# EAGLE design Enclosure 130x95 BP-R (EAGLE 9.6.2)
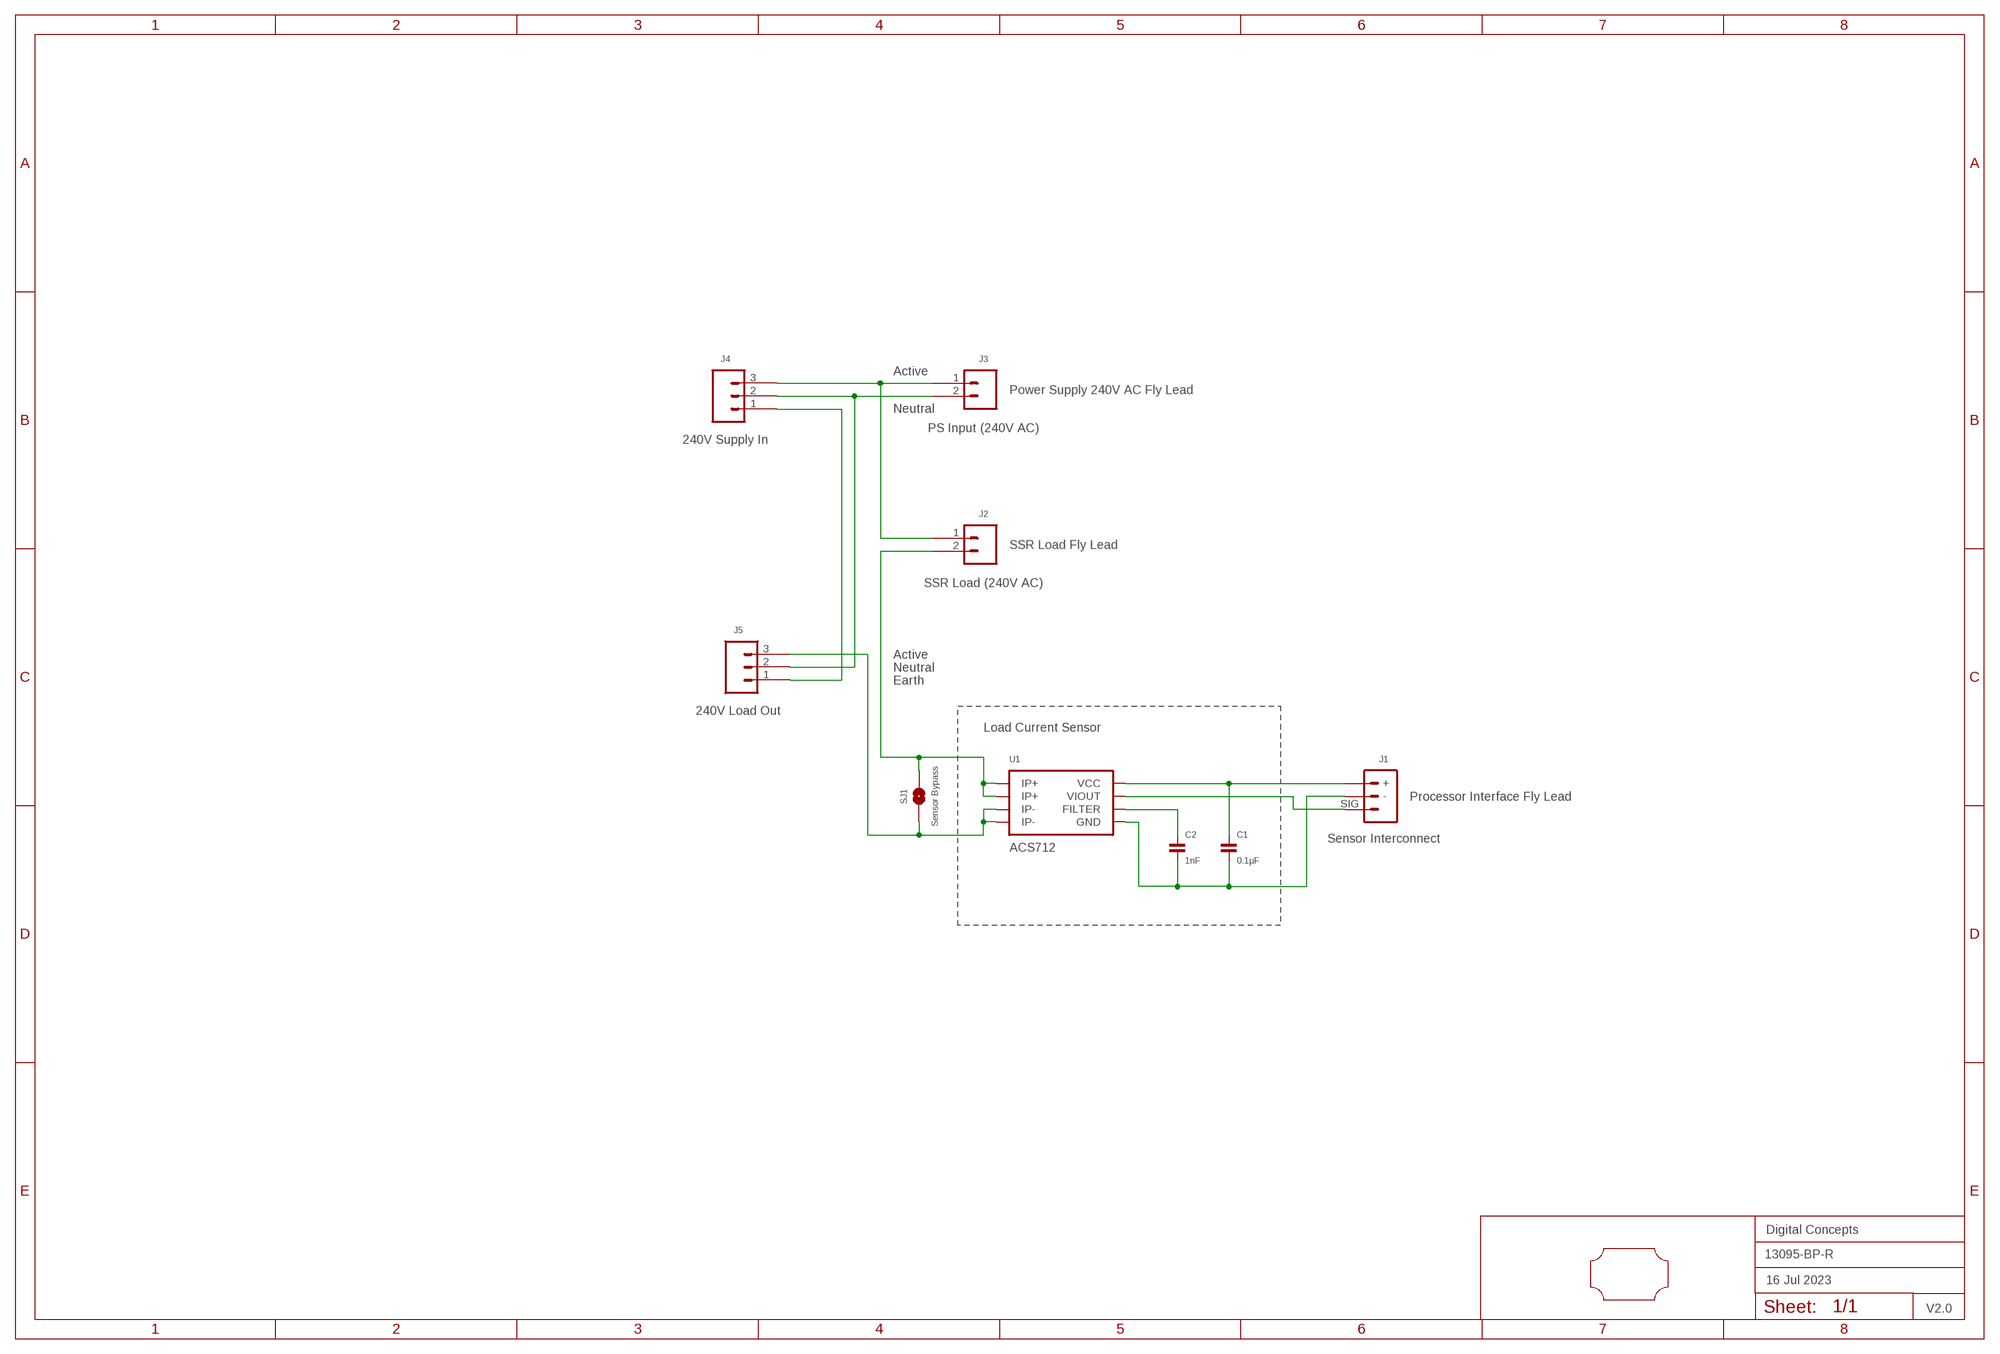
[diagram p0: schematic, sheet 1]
FRAME2 (A3L-LOC): DATE: 16 Jul 2023; OWNER: Digital Concepts; TITLE: 13095-BP-R; VERSION: V2.0

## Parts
C1  0.1µF  CAPACITOR-0805  [C0805]
C2  1nF  CAPACITOR-0805  [C0805]
J1  Sensor Interconnect  JST-PH2.0-3-HORIZONTAL  [JST-PH2.0-3-HORIZONTAL-SIG]
J2  SSR Load (240V AC)  TERMINAL_SCREW_2P_VERTICAL  [TERMINAL-SCREW-2P]
J3  PS Input (240V AC)  JST-XH2.54-2-HORIZONTAL  [JST-XH2.4-2-HORIZONTAL]
J4  240V Supply In  TERMINAL_SCREW_3P_VERTICAL  [TERMINAL-SCREW-3P]
J5  240V Load Out  TERMINAL_SCREW_3P_VERTICAL  [TERMINAL-SCREW-3P]
SJ1  Sensor Bypass  SJ  [SJ]
U1  ACS712  [SOIC-8]
U$1  PCB-OUTLINE-130X95-MAX-RC-H2  [PROTO-130X95-OUTLINE-MAX-RC-H2]

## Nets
ACTIVE_IN: J2.1 J3.1 J4.3
ACTIVE_OUT: J2.2 SJ1.2 U1.P$1(IP+) U1.P$2(IP+)
EARTH: J4.1 J5.1
N$19: J5.3 SJ1.1 U1.P$3(IP-) U1.P$4(IP-)
N$20: C1.2 C2.2 J1.- U1.P$5(GND)
N$22: J1.SIG U1.P$7(VIOUT)
N$23: C1.1 J1.+ U1.P$8(VCC)
N$24: C2.1 U1.P$6(FILTER)
NEUTRAL: J3.2 J4.2 J5.2

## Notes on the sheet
- Active
- Power Supply 240V AC Fly Lead
- Neutral
- SSR Load Fly Lead
- Active
- Neutral
- Earth
- Load Current Sensor
- Processor Interface Fly Lead

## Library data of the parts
C1 C2 = digitalconcepts:CAPACITOR-0805: 0805 Capacitor
J1 = digitalconcepts:JST-PH2.0-3-HORIZONTAL: PH2.0 3P Horizontal Connector
J2 = digitalconcepts:TERMINAL_SCREW_2P_VERTICAL: PCB Mount Screw-Type Terminal 2P
J3 = digitalconcepts:JST-XH2.54-2-HORIZONTAL: XH2.54 2P Horizontal Connector
J4 J5 = digitalconcepts:TERMINAL_SCREW_3P_VERTICAL: PCB Mount Screw-Type Terminal 3P
SJ1 = digitalconcepts:SJ: Solder Jumper
U1 = digitalconcepts:ACS712: ACS712 Hall-Effect-Based Linear Current Sensor IC
U$1 = digitalconcepts:PCB-OUTLINE-130X95-MAX-RC-H2: PCB Eagle Max-Right-Cropped outline for 130 x 95 enclosure (Horizontal format)

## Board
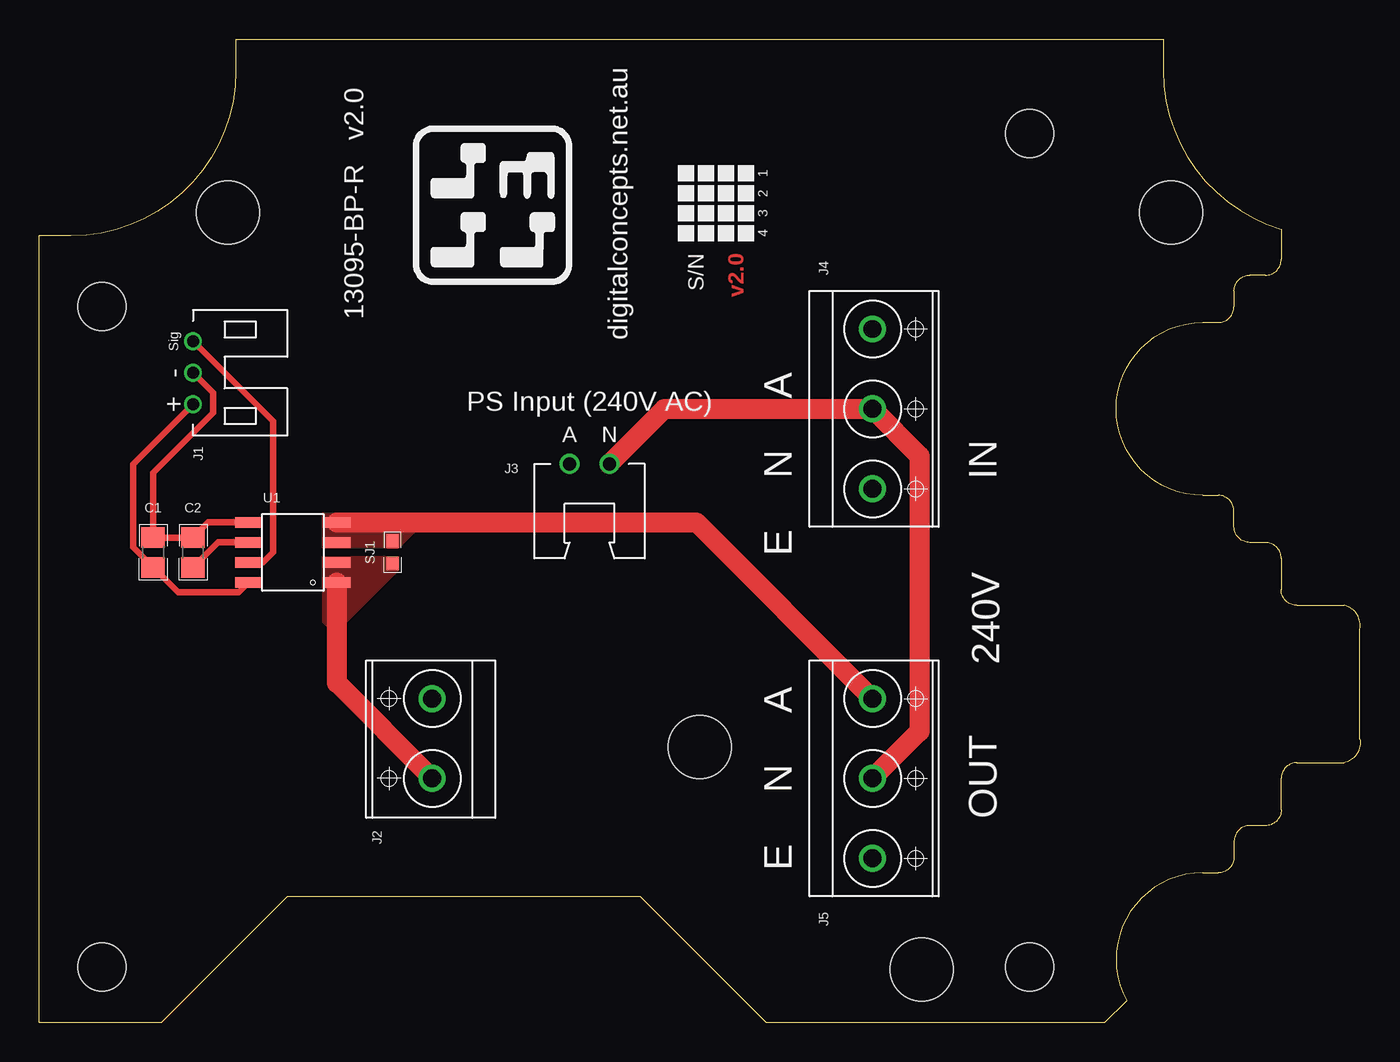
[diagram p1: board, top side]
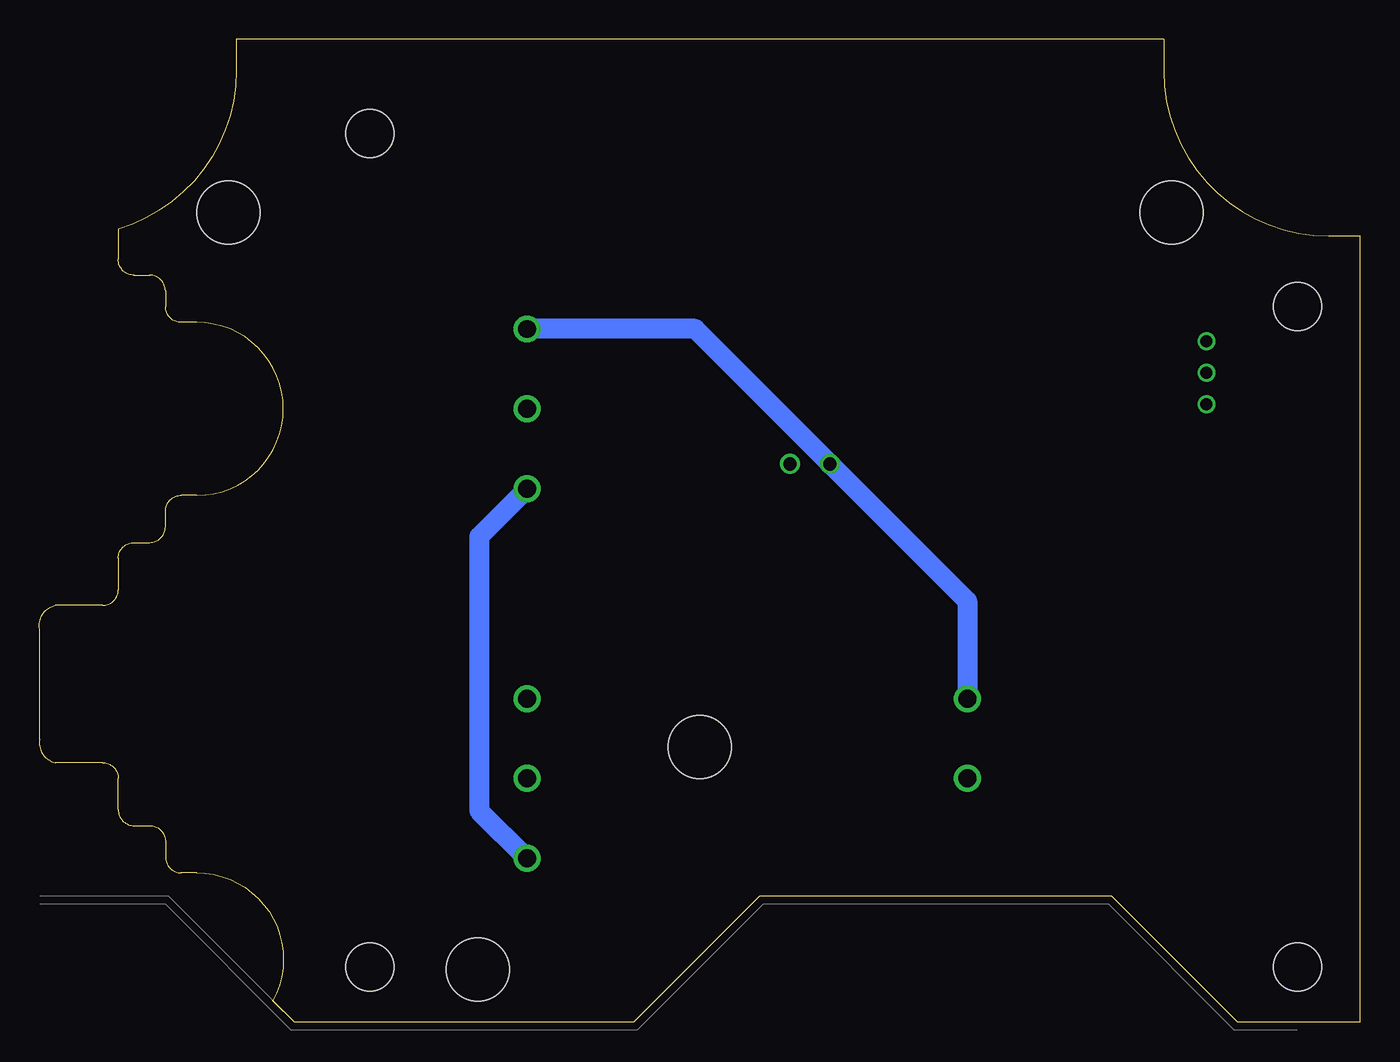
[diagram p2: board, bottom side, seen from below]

Size 84.02 x 62.5 mm. Coordinates in mm from the lower left corner, seen from the top.
Copper layers (1*16): Top 0.035mm / dielectric 1.5mm / Bottom 0.035mm
Design rules "default *": minimum track width 6mil, minimum drill 0.35mm, track to track 6mil, track to pad 6mil, pad to pad 6mil, via to via 6mil, smd to smd 6mil, copper to edge 6mil, drill to drill 6mil, minimum pad ring 1mil, minimum via ring 8mil, stop-mask expansion 4mil, vias tented up to drill 0mil, thermal gap 10mil

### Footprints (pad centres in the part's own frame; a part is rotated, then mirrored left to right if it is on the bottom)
C0805 = smd 1.3 x 1.5: 1 -0.95,0; 2 0.95,0
JST-PH2.0-3-HORIZONTAL-SIG = drill 0.75: + 2,0; - 0,0; SIG -2,0
TERMINAL-SCREW-2P = drill 1.143: 1 -2.58,0; 2 2.5,0
JST-XH2.4-2-HORIZONTAL = drill 0.85: 1 1.27,0; 2 -1.27,0
TERMINAL-SCREW-3P = drill 1.143: 1 -5.08,0; 2 0,0; 3 5.08,0
SJ = smd 0.864 x 0.762: 1 -0.711,0; 2 0.711,0
SOIC-8 = smd 0.65 x 1.75: P$1 -1.905,-2.8; P$2 -0.635,-2.8; P$3 0.635,-2.8; P$4 1.905,-2.8; P$5 1.905,2.8; P$6 0.635,2.8; P$7 -0.635,2.8; P$8 -1.905,2.8
PROTO-130X95-OUTLINE-MAX-RC-H2 = hole 3.048: -38,10; 21,21; 21,-32; -38,-32 | hole 4: 0,-18; -30,16; 30,16; 14.14,-32.14

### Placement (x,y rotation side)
C1  7.24,29.87 90 top
C2  9.78,29.87 90 top
J1  9.78,41.3 270 top
J2  25,18 270 top
J3  35,35.5 180 top
J4  53,39 90 top
J5  53,15.5 90 top
SJ1  22.48,29.87 270 top
U1  16.13,29.87 90 top
U$1  42,35.5 0 top

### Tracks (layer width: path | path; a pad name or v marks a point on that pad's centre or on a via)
ACTIVE_IN
  Bottom 1.27: J4.3 42.31,44.08 J3.1 25,26.77 J2.1
ACTIVE_OUT
  Top 1.27: J2.2 18.93,21.57 U1.P$1
  pour Top (no thermals): 18.04,29.62 22.86,29.62 22.86,28.73 19.18,25.04 18.42,25.04 18.04,25.42
EARTH
  Bottom 1.27: J4.1 56.04,30.88 56.04,13.46 J5.1
N$19
  Top 1.27: J5.3 41.8,31.77 U1.P$4
  pour Top (no thermals): 18.04,32.41 23.75,32.41 24.38,31.77 24.38,31.65 22.86,30.12 18.04,30.12
N$20
  Top 0.406: U1.P$5 10.73,31.77 C2.2 C1.2 7.24,34.95 11.05,38.76 11.05,40.03 J1.-
N$22
  Top 0.406: J1.SIG 14.86,38.22 14.86,29.87 14.23,29.23 U1.P$7
N$23
  Top 0.406: U1.P$8 12.7,27.33 8.83,27.33 C1.1 6.35,29.81 6.34,29.81 5.97,30.19 5.97,35.49 J1.+
N$24
  Top 0.406: C2.1 10.67,29.81 10.68,29.81 11.37,30.51 U1.P$6
NEUTRAL
  Top 1.27: J3.2 39.77,39 J4.2 56,36 56,18.5 J5.2

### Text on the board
Top: v2.0
tPlace: 1 | 13095-BP-R v2.0 | digitalconcepts.net.au | 2 | 3 | 4 | S/N
tNames: A | A | N | N | IN | E | 240V | A | N | OUT | E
